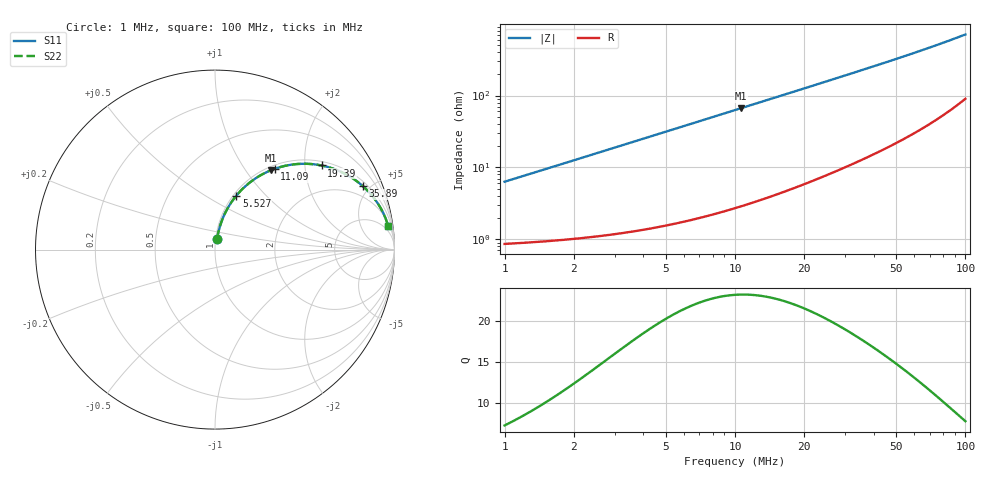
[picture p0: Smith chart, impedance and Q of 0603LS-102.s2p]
# MHz S MA R 50
!Freq  MagS11  AngS11  MagS21  AngS21  MagS12  AngS12  MagS22  AngS22
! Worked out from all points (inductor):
!   801 points, 1 MHz to 100 MHz, reference 50 ohm
!   read as one part in series: L = 997 nH near 1.023 MHz
!   highest Q = 23.2 at 10.59 MHz (marker M1), where L = 997 nH
!   S11 on the Smith chart (normalised r, x): 1 MHz: 1.02, +0.13; 5.527 MHz: 1.03, +0.69; 11.09 MHz: 1.06, +1.39; 19.39 MHz: 1.11, +2.44; 35.89 MHz: 1.26, +4.56; 100 MHz: 3, +14
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1  0.06255 78.6  0.9896 -3.6  0.9896 -3.6  0.06255 78.6
1.34122  0.08342 79.1  0.9876 -4.8  0.9876 -4.8  0.08342 79.1
1.717908  0.1064 78.8  0.9848 -6.1  0.9848 -6.1  0.1064 78.8
2.162719  0.1332 78.0  0.981 -7.6  0.981 -7.6  0.1332 78.0
2.676086  0.1638 76.8  0.9756 -9.4  0.9756 -9.4  0.1638 76.8
3.273407  0.1988 75.1  0.9683 -11.4  0.9683 -11.4  0.1988 75.1
3.935501  0.2366 73.2  0.9588 -13.7  0.9588 -13.7  0.2366 73.2
5.527134  0.3227 68.5  0.9312 -18.8  0.9312 -18.8  0.3227 68.5
7.807284  0.4322 61.9  0.8829 -25.6  0.8829 -25.6  0.4322 61.9
10.59254  0.5427 54.7  0.8168 -32.8  0.8168 -32.8  0.5427 54.7
11.09175  0.56 53.5  0.8047 -34.0  0.8047 -34.0  0.56 53.5
14.0443  0.6475 47.2  0.7343 -40.3  0.7343 -40.3  0.6475 47.2
17.57924  0.7254 41.0  0.6564 -46.4  0.6564 -46.4  0.7254 41.0
19.38653  0.7564 38.3  0.6202 -49.1  0.6202 -49.1  0.7564 38.3
26.0016  0.8357 30.6  0.509 -56.6  0.509 -56.6  0.8357 30.6
34.08003  0.8893 24.2  0.4108 -62.6  0.4108 -62.6  0.8893 24.2
35.89219  0.8975 23.1  0.393 -63.6  0.393 -63.6  0.8975 23.1
42.65795  0.9209 19.7  0.3371 -66.8  0.3371 -66.8  0.9209 19.7
50.69907  0.9388 16.6  0.2865 -69.5  0.2865 -69.5  0.9388 16.6
67.22023  0.9588 12.4  0.2154 -72.8  0.2154 -72.8  0.9588 12.4
83.65656  0.9683 9.7  0.1695 -74.4  0.1695 -74.4  0.9683 9.7
100  0.9732 7.8  0.1374 -74.9  0.1374 -74.9  0.9732 7.8
